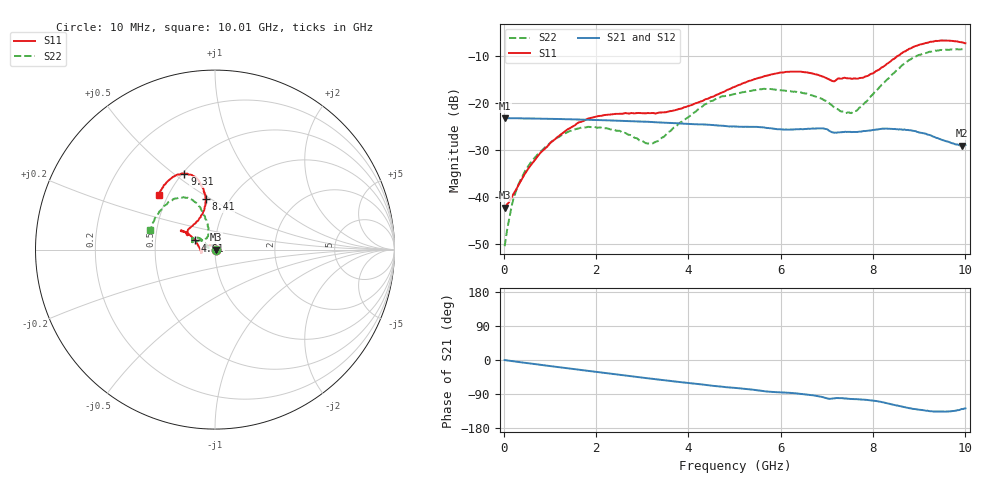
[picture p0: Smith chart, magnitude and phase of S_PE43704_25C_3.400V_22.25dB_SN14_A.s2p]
! Device ID: PE43704
! Dir: z:\PE43704\PE43704_Char_1_20130516\PE43704\AMB\3p400V\22p25dB
! Serial: 14
! Insertion: A
! Impedance: 50 ohm
! Temp: Amb
! VDD: 3.400V
! Attenuation Step: 22.25dB
! IDD: 1.140146e-01mA
#  Hz  S  RI  R  50
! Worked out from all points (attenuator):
!   401 points, 10 MHz to 10.01 GHz, reference 50 ohm
!   highest |S21| = -23.19 dB at 10 MHz (marker M1); lowest = -29.1 dB at 9.935 GHz (marker M2)
!   lowest |S11| = -42.4 dB at 10 MHz (marker M3), VSWR 1.02, Z = 50.8 + j0.0388 ohm
!   |S11| at or under -10 dB: start of sweep to 8.527 GHz
!   |S22| runs from -50.6 to -8.5 dB; largest |S21 - S12| = 0.00084
!   S11 on the Smith chart (normalised r, x): 10 MHz: 1.02, +0.00; 4.61 GHz: 0.79, +0.08; 8.41 GHz: 0.77, +0.47; 9.31 GHz: 0.51, +0.55; 10.01 GHz: 0.45, +0.33
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1e7  0.00761 0.000383  0.0692 -0.000187  0.0693 -0.00023  0.00293 0.00043
2.35e8  0.00553 0.00993  0.0688 -0.00467  0.0688 -0.0047  0.0014 0.0106
5.1e8  -0.00237 0.0194  0.0679 -0.00986  0.0679 -0.00985  -0.00592 0.0199
1.06e9  -0.0316 0.0239  0.065 -0.0198  0.065 -0.0197  -0.0314 0.024
1.685e9  -0.0632 0.00723  0.0597 -0.03  0.0597 -0.0299  -0.0545 0.00767
2.485e9  -0.0751 -0.016  0.0507 -0.0405  0.0507 -0.0406  -0.0504 -0.00662
3.11e9  -0.0768 -0.0159  0.0423 -0.0471  0.0423 -0.0471  -0.0368 0.00503
3.36e9  -0.0787 -0.00971  0.0384 -0.049  0.0386 -0.049  -0.0373 0.014
4.31e9  -0.0999 0.035  0.0253 -0.0536  0.0253 -0.0537  -0.0748 0.0556
4.61e9  -0.1119 0.0513  0.0207 -0.0542  0.0207 -0.0541  -0.0908 0.0647
5.01e9  -0.1313 0.0729  0.0159 -0.0541  0.0159 -0.054  -0.1089 0.0626
5.96e9  -0.182 0.1054  0.00438 -0.0525  0.00451 -0.0524  -0.1278 0.0522
6.685e9  -0.1824 0.1005  -0.00281 -0.0535  -0.00295 -0.0532  -0.1131 0.0431
7.135e9  -0.1494 0.0849  -0.00966 -0.0477  -0.00971 -0.0478  -0.0782 0.0502
7.535e9  -0.1282 0.1301  -0.0108 -0.0479  -0.0108 -0.0479  -0.0457 0.0636
7.86e9  -0.0876 0.1731  -0.0133 -0.0488  -0.0134 -0.049  -0.0363 0.0973
8.36e9  -0.0524 0.2683  -0.0229 -0.0481  -0.023 -0.0481  -0.0548 0.1802
8.41e9  -0.0529 0.2821  -0.0241 -0.0472  -0.024 -0.0474  -0.0614 0.191
8.835e9  -0.0866 0.3775  -0.0314 -0.0403  -0.0312 -0.0404  -0.1193 0.271
9.31e9  -0.1707 0.4225  -0.0316 -0.0305  -0.0321 -0.0306  -0.2173 0.2851
9.935e9  -0.3022 0.3295  -0.0222 -0.0272  -0.0227 -0.0269  -0.3501 0.1405
1.001e10  -0.3134 0.3037  -0.0218 -0.0282  -0.022 -0.0281  -0.3595 0.1109
